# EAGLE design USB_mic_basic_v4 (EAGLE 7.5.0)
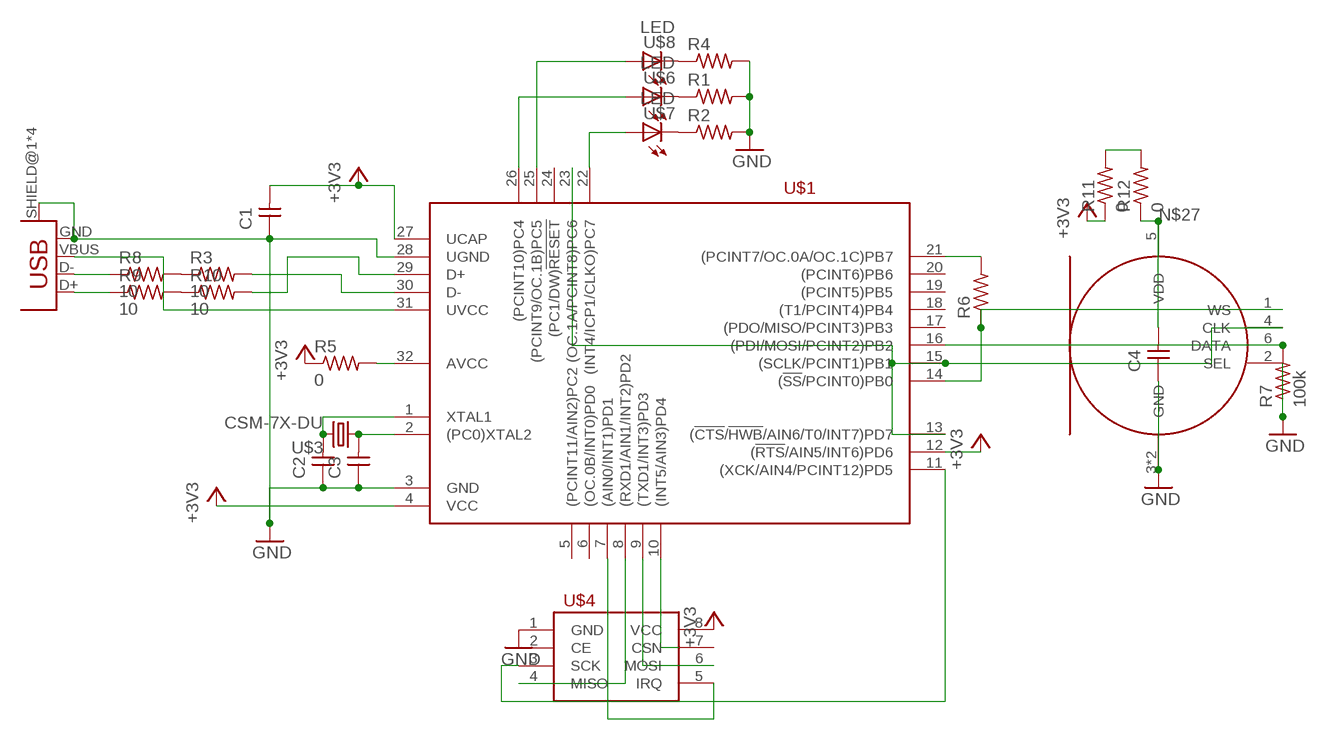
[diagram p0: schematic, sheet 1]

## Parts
C1  CAP-UNPOLARIZEDFAB  [C1206FAB]
C2  CAP-UNPOLARIZEDFAB  [C1206FAB]
C3  CAP-UNPOLARIZEDFAB  [C1206FAB]
C4  CAP-UNPOLARIZEDFAB  [C1206FAB]
R1  RES-US1206FAB  [R1206FAB]
R2  RES-US1206FAB  [R1206FAB]
R3  10  RES-US1206FAB  [R1206FAB]
R4  RES-US1206FAB  [R1206FAB]
R5  0  RES-US1206FAB  [R1206FAB]
R6  RES-US1206FAB  [R1206FAB]
R7  100k  RES-US1206FAB  [R1206FAB]
R8  10  RES-US1206FAB  [R1206FAB]
R9  10  RES-US1206FAB  [R1206FAB]
R10  10  RES-US1206FAB  [R1206FAB]
R11  0  RES-US1206FAB  [R1206FAB]
R12  0  RES-US1206FAB  [R1206FAB]
U$1  ATMEGA16U2-TQ  [TQFP32-08THIN]
U$2  USB_MINIB  [USB_MINIB]
U$3  CSM-7X-DU  [CSM-7X-DU]
U$4  NRF24L01+  [2X04_THRU]
U$5  MEMS_MIC_SPH0645LM4H-BI2S  [MIC_BOTTOM_PORT]
U$6  LED  [LED1206]
U$7  LED  [LED1206]
U$8  LED  [LED1206]

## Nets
+3V3: C1.2 R5.1 R11.1 U$1.4(VCC) U$1.12((!RTS!/AIN5/INT6)PD6) U$1.27(UCAP) U$4.8(VCC)
GND: C1.1 C2.1 C3.1 C4.1 R1.2 R2.2 R4.2 R7.1 U$1.3(GND) U$1.28(UGND) U$2.GND U$2.SHIELD@1(SHIELD) U$2.SHIELD@2(SHIELD) U$2.SHIELD@3(SHIELD) U$2.SHIELD@4(SHIELD) U$4.1(GND) U$5.2(SEL) U$5.3(GND) U$5.P$1(GND)
N$1: R3.2 U$1.30(D-)
N$2: R10.2 U$1.29(D+)
N$3: U$1.31(UVCC) U$2.VBUS
N$4: U$1.25((PCINT9/OC.1B)PC5) U$8.1(A)
N$5: U$1.26((PCINT10)PC4) U$6.1(A)
N$6: C2.2 U$1.1(XTAL1) U$3.2
N$7: C3.2 U$1.2((PC0)XTAL2) U$3.1
N$8: R1.1 U$6.2(C)
N$9: R6.1 U$1.14((!SS!/PCINT0)PB0) U$5.1(WS)
N$10: U$1.13((!CTS!/!HWB!/AIN6/T0/INT7)PD7) U$1.15((SCLK/PCINT1)PB1) U$1.23((OC.1A/PCINT8)PC6) U$5.4(CLK)
N$11: R7.2 U$1.16((PDI/MOSI/PCINT2)PB2) U$5.6(DATA)
N$12: U$1.7((AIN0/INT1)PD1) U$4.5(IRQ)
N$13: U$1.22((INT4/ICP1/CLKO)PC7) U$7.1(A)
N$14: U$1.9((TXD1/INT3)PD3) U$4.6(MOSI)
N$15: R2.1 U$7.2(C)
N$16: U$1.8((RXD1/AIN1/INT2)PD2) U$4.4(MISO)
N$17: R8.1 U$2.D-
N$18: R4.1 U$8.2(C)
N$19: U$1.11((XCK/AIN4/PCINT12)PD5) U$4.3(SCK)
N$20: R5.2 U$1.32(AVCC)
N$21: R9.1 U$2.D+
N$22: R3.1 R8.2
N$23: R9.2 R10.1
N$24: U$1.10((INT5/AIN3)PD4)
N$25: R6.2 U$1.21((PCINT7/OC.0A/OC.1C)PB7)
N$26: R11.2 R12.2
N$27: C4.2 R12.1 U$5.5(VDD)
Unconnected: U$1.5((PCINT11/AIN2)PC2) U$1.6((OC.0B/INT0)PD0) U$1.17((PDO/MISO/PCINT3)PB3) U$1.18((T1/PCINT4)PB4) U$1.19((PCINT5)PB5) U$1.20((PCINT6)PB6) U$1.24((PC1/DW)!RESET) U$4.2(CE) U$4.7(CSN)

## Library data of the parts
C1-C4 = fab:CAP-UNPOLARIZED
R1-R12 = fab:RES-US: Resistor (US Symbol)
U$1 = fab:ATMEGA16U2
U$2 = fab:USB_MINIB
U$3 = crystal:CSM-7X-DU: SMD CRYSTAL; OC_FARNELL: unknown; OC_NEWARK: unknown
U$4 = fab:NRF24L01+: nRF24L01+ 2.4GHz Wireless Transceiver module
U$5 = fab:MEMS_MIC_SPH0645LM4H-B
U$6-U$8 = fab:LED: LED

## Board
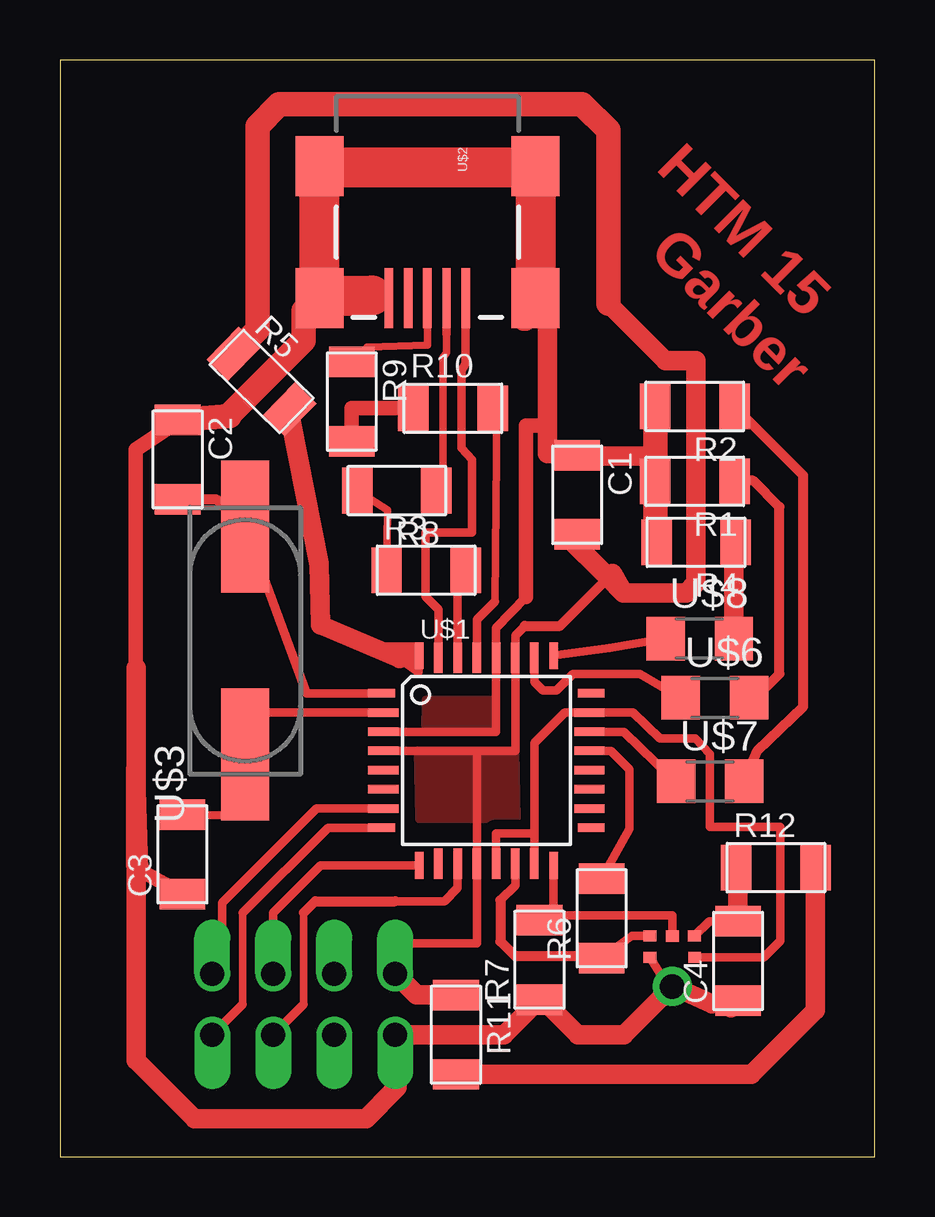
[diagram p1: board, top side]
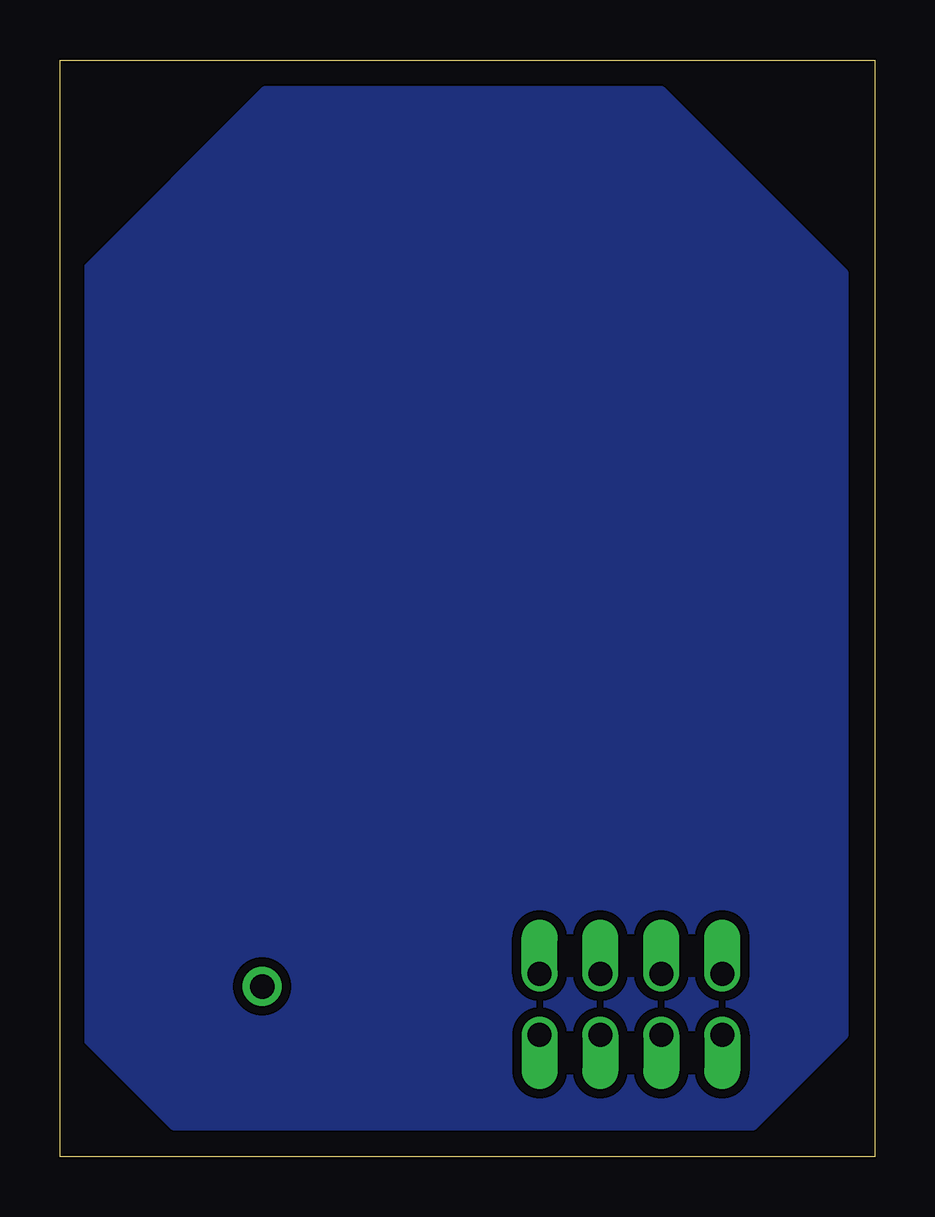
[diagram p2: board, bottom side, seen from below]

Size 33.96 x 45.71 mm. Coordinates in mm from the lower left corner, seen from the top.
Outline: 0,0 33.96,0 33.96,45.71 0,45.71 0,0
Copper layers (1*16): Top 0.035mm / dielectric 1.5mm / Bottom 0.035mm
Design rules "fab": minimum track width 0.3mm, minimum drill 32mil, track to track 0.397mm, track to pad 0.397mm, pad to pad 0.397mm, via to via 0.397mm, smd to smd 0.315mm, copper to edge 40mil, drill to drill 16mil, minimum pad ring 10mil, minimum via ring 8mil, stop-mask expansion 4mil, vias tented up to drill 0mil, thermal gap 10mil

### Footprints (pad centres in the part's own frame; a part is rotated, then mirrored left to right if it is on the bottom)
C1206FAB = smd 1.27 x 1.905: 1 -1.651,0; 2 1.651,0
R1206FAB = smd 1.27 x 1.905: 1 -1.651,0; 2 1.651,0
TQFP32-08THIN = smd 1.118 x 0.356: 1 -4.369,2.8; 8 -4.369,-2.8; 17 4.369,-2.8; 24 4.369,2.8 | smd 1.27 x 0.356: 2 -4.293,2; 3 -4.293,1.2; 4 -4.293,0.4; 5 -4.293,-0.4; 6 -4.293,-1.2; 7 -4.293,-2; 18 4.293,-2; 19 4.293,-1.2; 20 4.293,-0.4; 21 4.293,0.4; 22 4.293,1.2; 23 4.293,2 | smd 0.356 x 1.118: 9 -2.8,-4.369; 16 2.8,-4.369; 25 2.8,4.369; 32 -2.8,4.369 | smd 0.356 x 1.27: 10 -2,-4.293; 14 1.2,-4.293; 15 2,-4.293; 26 2,4.293; 27 1.2,4.293; 31 -2,4.293 | smd 0.35 x 1.27: 11 -1.2,-4.293; 12 -0.4,-4.293; 13 0.4,-4.293; 28 0.4,4.293; 29 -0.4,4.293; 30 -1.2,4.293
USB_MINIB = smd 2.5 x 0.35: D+ 3.77,0; D- 3.77,0.8; GND 3.77,-1.6; ID 3.77,-0.8; VBUS 3.77,1.6 | smd 2.5 x 2: SHIELD@1 -1.73,-4.5; SHIELD@2 -1.73,4.5; SHIELD@3 3.77,4.5; SHIELD@4 3.77,-4.5
CSM-7X-DU = smd 5.5 x 2: 1 -4.75,0; 2 4.75,0
2X04_THRU = drill 1 pad 1.27 offset: 1 -1.27,3.81; 2 -1.27,1.27; 3 -1.27,-1.27; 4 -1.27,-3.81; 5 1.27,-3.81; 6 1.27,-1.27; 7 1.27,1.27; 8 1.27,3.81
MIC_BOTTOM_PORT = smd 0.54 x 0.46: 1 -0.929,2.106; 2 -0.931,1.221; 4 0.931,1.22; 5 0.93,2.105; 6 0,2.102 | smd 1.624 x 1.624: 3 0,0 | drill 1.024 pad 1.624: P$1 0,0
LED1206 = smd 1.6 x 1.803: 1 -1.422,0; 2 1.422,0

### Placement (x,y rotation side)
C1  21.56,27.58 270 top
C2  4.9,29.06 270 top
C3  5.11,12.6 90 top
C4  28.27,8.15 90 top
R1  26.47,28.14 180 top
R2  26.47,31.27 180 top
R3  15.27,24.43 0 top
R4  26.52,25.6 180 top
R5  8.41,32.31 315.6 top
R6  22.58,9.93 90 top
R7  19.99,8.2 90 top
R8  14.05,27.76 180 top
R9  12.17,31.47 270 top
R10  16.38,31.19 0 top
R11  16.51,5.08 270 top
R12  29.84,12.04 0 top
U$1  17.78,16.51 0 top
U$2  15.32,39.55 270 top
U$3  7.72,21.51 90 top
U$4  10.16,6.35 90 bottom
U$5  25.53,7.09 0 top
U$6  27.3,19.13 0 top
U$7  27.1,15.65 0 top
U$8  26.67,21.59 0 top

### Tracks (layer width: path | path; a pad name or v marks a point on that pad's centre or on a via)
+3V3
  Top 0.356: 19.38,22.12 18.98,21.72 U$1.27 18.98,16.91 17.38,16.91 | 17.38,16.91 U$1.4 | 17.38,16.91 U$1.12 17.38,8.89 13.97,8.89 U$4.8
  Top 0.406: 19.38,22.12 20.85,22.12 22.86,24.13
  Top 0.813: 23.04,24.31 23.5,23.5 | 23.5,23.5 26.11,23.5 26.52,23.9 26.52,33.17 25.25,33.17 22.86,35.56 | C1.2 21.03,25.96 22.86,24.13 23.5,23.5 | R11.1 14.86,6.73 U$4.8
  Top 1.016: 22.86,35.56 22.86,42.77 21.77,43.87 9.14,43.87 8.23,42.95 8.23,34.47 R5.1
  pour Top: 14.91,16.94 14.96,14.05 19.05,14.05 19,16.94
BACK
  pour Bottom: 33.02,36.83 33.02,5.08 29.21,1.27 5.08,1.27 1.27,5.08 1.27,36.83 8.89,44.45 25.4,44.45
GND
  Top 0.305: U$2.SHIELD@3 19.13,35.09 | 13.97,2.79 14.05,2.87 14.05,2.9
  Top 0.356: U$2.GND U$2.SHIELD@4 | U$1.3 17.78,17.71 17.63,17.7 18.18,17.7 U$1.28 18.18,22.04 19.43,23.32 | 19.13,35.09 19.46,34.72 | U$2.SHIELD@2 19.82,41.22 19.13,41.22 | 10.9,41.22 10.9,41.28 U$2.SHIELD@1 | U$5.2 25.4,7.01 26.11,6.84
  Top 0.61: C3.1 3.38,11.91 3.15,19.43 3.15,29.46 5.08,30.73 C2.1 | 19.33,34.82 19.46,34.72 | 19.43,23.32 19.43,30.48 20.32,30.48
  Top 0.813: 27.96,6.2 C4.1 27.18,6.38 26.11,6.84 U$5.P$1 23.52,5.08 21.59,5.08 20.12,6.55 R7.1 18.52,5.08 U$4.1 14.1,4.95 14.1,4.93 14.05,4.88 14.05,2.9 | 19.33,34.82 19.33,35.56 20.32,35.56 20.32,30.48 20.32,29.31 C1.1 21.03,29.21 24.82,29.21 | 13.97,2.79 12.75,1.57 5.61,1.57 3.17,4.01 3.17,20.37 3.15,12.14 3.38,11.91
  Top 1.016: C2.1 7.04,30.86 | 7.04,30.86 7.07,30.86 | R2.2 24.82,29.21 R1.2 24.82,25.65 R4.2 | 7.04,30.86 7.04,30.89 10.16,34.01 10.16,35.26 10.74,35.84 10.81,35.78 U$2.SHIELD@4
  Top 1.676: U$2.SHIELD@1 U$2.SHIELD@4 10.93,35.89 13.01,35.89 | U$2.SHIELD@2 U$2.SHIELD@3 | 19.58,41.22 19.13,41.22 10.9,41.22 10.9,41.2
  pour Top: 15.21,17.7 15.24,19.05 18.14,19.05 18.16,17.68
N$1
  Top 0.356: R3.2 16.58,24.3 U$1.30
N$2
  Top 0.305: 18.14,23.14 18.21,31.19 R10.2
  Top 0.356: 18.14,23.14 17.38,22.38 U$1.29
N$3
  Top 0.356: U$2.VBUS 16.92,33.05 16.74,32.77 16.74,29.54 17.17,29.06 17.17,26.01 15.24,26.01 15.24,23.34 15.78,22.8 U$1.31
N$4
  Top 0.356: U$1.25 22.91,21.21 U$8.1
N$5
  Top 0.356: U$1.26 19.78,19.79 20.14,19.43 20.7,19.43 21.39,20.12 24.18,20.12 U$6.1
N$6
  Top 0.356: U$1.1 10.29,19.31 U$3.2
  Top 0.406: C2.2 6.51,27.4 U$3.2
N$7
  Top 0.356: U$1.2 7.62,18.51 U$3.1 7.77,14.23 C3.2
N$8
  Top 0.406: U$6.2 28.93,19.05 30,20.12 30,27.08 28.91,28.17 28.14,28.17 R1.1
N$9
  Top 0.356: R6.1 23.85,9.19 U$5.1 | U$1.14 18.98,11.31 18.36,10.69
  Top 0.406: 18.36,10.69 18.36,8.97 18.97,8.36 22.15,8.36 R6.1
N$10
  Top 0.356: 19.78,13.46 19.78,17.24 21.05,18.51 U$1.23 23.88,18.51 25.02,17.42 26.49,17.42 27.1,16.79 27.1,13.74 30.02,13.74 30.02,8.99 29.34,8.31 U$5.4 | 19.78,13.46 U$1.15 | U$1.13 18.18,13.46 19.78,13.46
N$11
  Top 0.356: U$1.16 20.58,10.06 25.53,10.06 U$5.6
  Top 0.406: 20.58,10.06 20.07,10.01 R7.2
N$12
  Top 0.356: U$4.5 6.76,9.5 6.76,10.57 10.7,14.51 U$1.7
N$13
  Top 0.356: U$1.22 23.52,17.71 25.48,15.8 U$7.1
N$14
  Top 0.356: U$4.6 8.89,10.16 10.87,12.14 U$1.9
N$15
  Top 0.406: U$7.2 29.08,16.92 30.99,18.75 30.99,28.4 R2.1
N$16
  Top 0.305: 7.62,6.35 7.62,10.16
  Top 0.356: U$4.4 7.62,6.35 | 7.62,10.16 11.17,13.71 U$1.8
N$17
  Top 0.305: 16.12,34.28 16.12,33.52 15.98,33.3 15.98,27.89 15.79,27.18 R8.1
  Top 0.356: U$2.D- 16.12,34.28
N$18
  Top 0.813: U$8.2 28.09,25.6 R4.1
N$19
  Top 0.305: 10.16,6.35 10.16,10.16
  Top 0.356: U$4.3 10.16,6.35 | 13.18,10.64 13.97,10.64 16.03,10.64 16.58,11.2 U$1.11
  Top 0.406: 10.16,10.16 10.64,10.64 13.97,10.64
N$20
  Top 0.305: 14.15,20.75 14.81,20.68 13.41,21.13
  Top 0.356: 14.15,20.75 14.96,20.19 U$1.32
  Top 0.61: 13.41,21.13 14.83,21.13
  Top 0.813: R5.2 9.63,30.61 10.79,24.7 10.86,22.16 14.15,20.75
N$21
  Top 0.305: U$2.D+ 15.32,33.83 12.8,33.73 12.78,33.12 R9.1
N$22
  Top 0.305: R3.1 13.66,26.95 R8.2
N$23
  Top 0.61: R9.2 12.17,31.19 R10.1
N$25
  Top 0.356: R6.2 23.75,13.66 23.75,16.13 22.97,16.91 U$1.21
N$26
  Top 0.813: R11.2 28.83,3.43 31.5,6.1 R12.2
N$27
  Top 0.356: C4.2 27.07,9.8 U$5.5
  Top 0.813: R12.1 28.27,11.96 C4.2

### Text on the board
Top: HTM 15 | Garber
